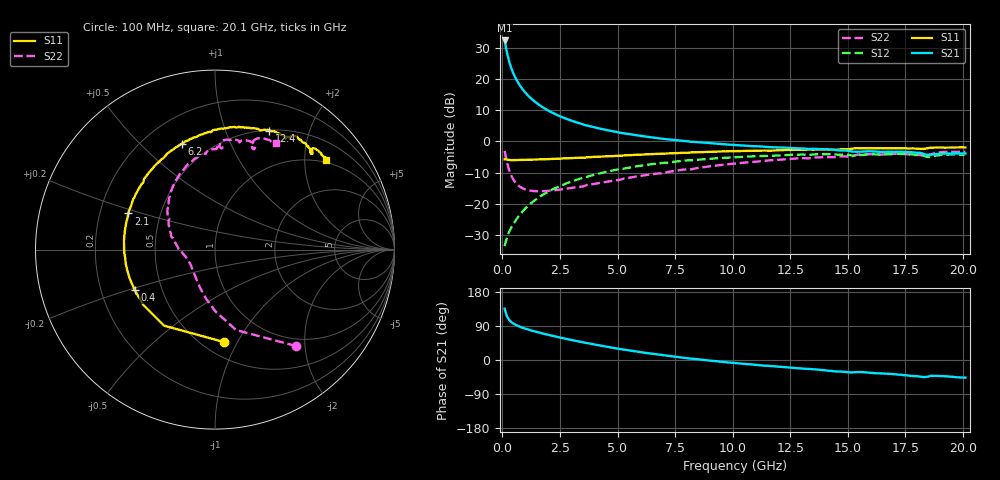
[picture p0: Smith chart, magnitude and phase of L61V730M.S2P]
!  Infineon Technologies AG
! BFR380L3 , PF131585-7, No.6, Th 09.10.01, soldered on pcb-board, measured with PP GSG850
!  Vce=1.75 V,  Ic=30.0 mA
! Common Emitter S-Parameters:  15. November 2001
#  GHz  S  MA  R  50
! f  S11  S21  S12  S22
! GHz  Mag  Ang  Mag  Ang  Mag  Ang  Mag  Ang
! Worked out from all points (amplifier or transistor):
!   201 points, 100 MHz to 20.1 GHz, reference 50 ohm
!   highest |S21| = 32.3 dB at 100 MHz (marker M1)
!   |S21| within 3 dB of that: start of sweep to 177.9 MHz
!   unconditionally stable (mu >= 1): 1.163 GHz to 4.377 GHz
!   at 3.4 GHz: K = 1.02, MAG = 8.0 dB, |S12| = -11.9 dB
!   at 10.1 GHz: K = 0.97, MSG = 2.0 dB, |S12| = -5.1 dB
!   at 20.1 GHz: K = 0.99, MSG = 0.2 dB, |S12| = -4.2 dB
!   S11 on the Smith chart (normalised r, x): 100 MHz: 0.63, -0.88; 400 MHz: 0.35, -0.21; 2.1 GHz: 0.32, +0.18; 6.2 GHz: 0.35, +0.68; 12.4 GHz: 0.51, +1.43; 20.1 GHz: 0.92, +2.54
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0.1  0.5171 -84.6  41.01 135.5  0.0211 60.4  0.7006 -50.0
0.2  0.5099 -123.8  26.32 115.3  0.02894 55.9  0.4633 -75.3
0.3  0.5044 -142.4  18.76 105.6  0.03608 57.0  0.3431 -89.8
0.4  0.5009 -153.5  14.46 99.7  0.04227 59.2  0.2776 -100.3
0.5  0.5015 -160.8  11.73 95.4  0.04886 61.4  0.2384 -108.7
0.6  0.5025 -166.5  9.852 92.2  0.05586 63.2  0.2135 -115.5
0.7  0.5037 -171.1  8.5 89.4  0.06287 64.3  0.1965 -121.5
0.9  0.5055 -177.8  6.658 84.7  0.07725 66.0  0.1761 -130.9
1.1  0.5075 177.0  5.489 80.8  0.09186 66.5  0.1669 -138.5
1.4  0.5115 170.2  4.348 75.6  0.1138 66.4  0.1602 -147.0
1.7  0.5157 164.3  3.609 70.8  0.1359 65.6  0.1599 -153.7
2.1  0.5227 157.3  2.959 64.9  0.1648 63.7  0.1636 -160.6
2.7  0.5356 148.2  2.35 56.7  0.2071 60.2  0.1739 -169.4
3.5  0.5477 137.1  1.866 46.6  0.2623 54.9  0.19 -178.0
4.8  0.5821 121.5  1.448 32.2  0.3426 45.7  0.2345 167.1
6.2  0.6188 107.3  1.197 19.0  0.4181 35.7  0.2888 153.0
6.8  0.6326 101.5  1.117 13.9  0.4459 31.2  0.3071 146.7
10.1  0.6974 77.6  0.8737 -8.1  0.5575 9.8  0.4427 119.5
12.4  0.7281 65.6  0.7896 -19.6  0.6066 -4.1  0.5207 101.8
13.5  0.7371 60.4  0.7602 -24.7  0.6169 -10.3  0.5464 94.8
16.8  0.7722 48.3  0.6839 -36.1  0.6222 -25.7  0.6288 75.4
20.1  0.7976 38.9  0.6415 -46.4  0.6163 -39.0  0.6821 60.1
